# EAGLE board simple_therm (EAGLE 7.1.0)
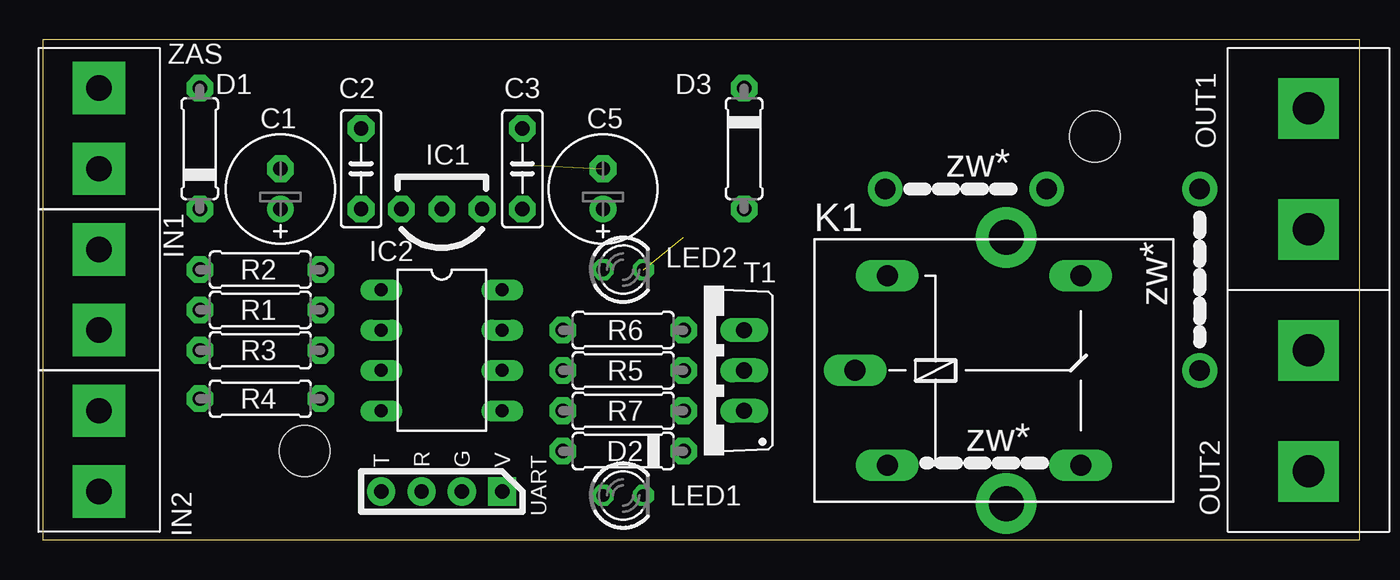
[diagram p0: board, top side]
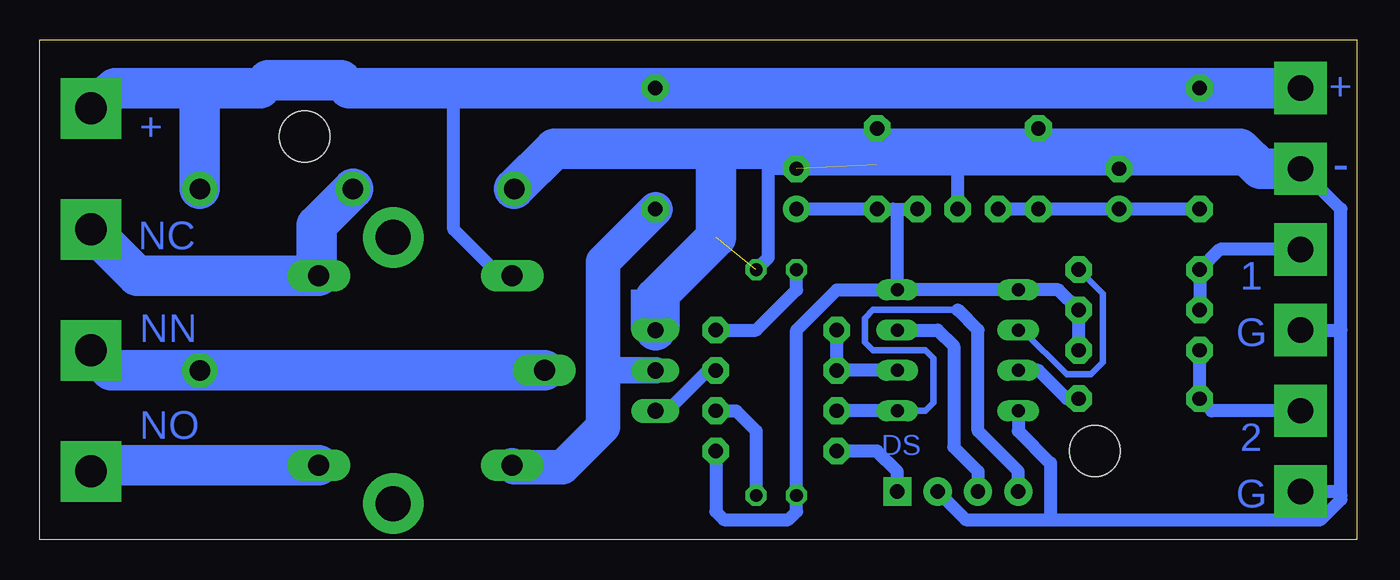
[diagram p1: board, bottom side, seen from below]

Size 82.98 x 31.49 mm. Coordinates in mm from the lower left corner, seen from the top.
Outline: 0,0 82.98,0 82.98,31.49 0,31.49 0,0
Copper layers (1*16): Top 0.035mm / dielectric 1.5mm / Bottom 0.035mm
Design rules "default": minimum track width 10mil, minimum drill 24mil, track to track 8mil, track to pad 8mil, pad to pad 8mil, via to via 8mil, smd to smd 8mil, copper to edge 40mil, drill to drill 8mil, minimum pad ring 10mil, minimum via ring 8mil, stop-mask expansion 4mil, vias tented up to drill 0mil, thermal gap 10mil
Holes 3.2 mm at 16.51,5.59 66.29,25.4

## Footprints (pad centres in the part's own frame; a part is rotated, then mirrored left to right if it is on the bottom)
E2,5-7 = drill 0.9 pad 1.676: + -1.27,0 | drill 0.9 pad 1.676 octagon: - 1.27,0
C050-025X075 = drill 0.9 pad 1.676 octagon: 1 -2.54,0; 2 2.54,0
0207/7 = drill 0.9 pad 1.676 octagon: 1 -3.81,0; 2 3.81,0
DIL08 = drill 0.813 long: 1 -3.81,-3.81; 2 -1.27,-3.81; 3 1.27,-3.81; 4 3.81,-3.81; 5 3.81,3.81; 6 1.27,3.81; 7 -1.27,3.81; 8 -3.81,3.81
ARK2/500 = drill 1.6 pad 3.302 square: 1 -2.54,0; 2 2.54,0
G5LE = drill 1.321 long: 1 -7.493,-5.969; 2 -7.493,5.969; O 4.699,5.969; P -9.525,0; S 4.699,-5.969
LED3MM = drill 0.813 octagon: A -1.27,0; K 1.27,0
ARK2/750 = drill 2 pad 3.81 square: 1 -3.81,0; 2 3.81,0
TO220BV = drill 1.016 long: D 0,-2.54; G -2.54,-2.54; S 2.54,-2.54
MOD09 = drill 0.9 pad 1.778 square: 1 0,-3.81 | drill 0.9 pad 1.778: 2 0,-1.27; 3 0,1.27; 4 0,3.81

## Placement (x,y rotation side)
C1  100uF  [E2,5-7]  14.99,22.1 90 top
C2  100nF  [C050-025X075]  20.07,23.37 90 top
C3  100nF  [C050-025X075]  30.23,23.37 90 top
C5  100uF  [E2,5-7]  35.31,22.1 90 top
D1  1N4007  [0207/7]  9.91,24.64 90 top
D2  1N4007  [0207/7]  36.58,5.59 180 top
D3  1N4007  [0207/7]  44.2,24.64 90 top
IC2  Attiny45  [DIL08]  25.15,11.94 270 top
IN1  ARK2ARK2/500  [ARK2/500]  3.56,15.75 270 top
IN2  ARK2ARK2/500  [ARK2/500]  3.56,5.59 270 top
K1  [G5LE]  60.71,10.67 0 top
LED1  [LED3MM]  36.58,2.79 0 top
LED2  [LED3MM]  36.58,17.02 0 top
OUT1  ARK2  [ARK2/750]  79.76,23.37 90 top
OUT2  ARK2  [ARK2/750]  79.76,8.13 90 top
R1  3k  [0207/7]  13.72,14.48 0 top
R2  3k  [0207/7]  13.72,17.02 0 top
R3  3k  [0207/7]  13.72,11.94 0 top
R4  3k  [0207/7]  13.72,8.89 0 top
R5  3k  [0207/7]  36.58,8.13 0 top
R6  3k  [0207/7]  36.58,13.21 0 top
R7  3k  [0207/7]  36.58,10.67 180 top
T1  N-MOSFET  [TO220BV]  41.66,10.67 90 top
UART  [MOD09]  25.15,3.05 90 top
ZAS  ARK2ARK2/500  [ARK2/500]  3.56,25.91 270 top

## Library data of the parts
C1-C3 C5 D1-D3 R1-R7 = rcl
IC2 = avr-7_2
IN1 IN2 OUT1 OUT2 ZAS = dimmer
K1 = relay; OC_FARNELL: unknown; OC_NEWARK: unknown
LED1 LED2 = led
T1 = transistor-power
UART = dslib_eagle 9_new

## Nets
GND: C1.- C2.2 C3.2 C5.- IC2.4 IN1.2 IN2.2 LED2.K T1.S UART.2 ZAS.2
IN1: IC2.2 R2.2
IN2: IC2.3 R4.2
N$1: K1.O OUT1.1
N$3: D2.2 UART.1
N$4: D3.1 K1.1 T1.D
N$5: IN1.1 R1.1 R2.1
N$6: LED2.A R6.2
N$8: IN2.1 R3.1 R4.1
N$11: LED1.K R5.2
N$14: R7.1 T1.G
N$16: K1.P OUT2.2
N$17: K1.S OUT2.1
OUT: IC2.6 R6.1 R7.2
RST: IC2.1
RX: IC2.7 UART.3
TX: IC2.5 R5.1 UART.4
V+: C1.+ C2.1 D1.1
VCC: D1.2 D3.2 K1.2 OUT1.2 ZAS.1
VDD: C3.1 C5.+ D2.1 IC2.8 LED1.A R1.2 R3.2

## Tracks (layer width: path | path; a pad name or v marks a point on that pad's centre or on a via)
GND  (via drill 1.3 pad 2.18)  (2 unrouted)
  Bottom 0.813: UART.2 24.64,1.27 19.3,1.27 | 19.3,1.27 2.29,1.27 1.02,2.54 1.02,2.79 | 1.02,2.79 1.02,13.21 | 1.02,13.21 1.02,20.83 ZAS.2 C1.- C5.- 37.08,23.37 37.08,17.78 LED2.K | IN1.2 1.02,13.21 | IN2.2 1.27,3.05 1.02,2.79 | IC2.4 21.34,6.86 19.3,4.83 19.3,1.27 | C2.2 20.07,23.37 29.97,23.37 30.23,23.62 C3.2
  Bottom 2.54: ZAS.2 6.1,23.37 7.37,24.64 50.55,24.64 v53.09,22.1 | 40.39,23.37 40.39,19.05 44.2,15.24 T1.S
IN1
  Bottom 0.406: IC2.2 21.08,13.21 18.29,10.41 16.76,10.41 16,11.18 16,15.49 R2.2
IN2
  Bottom 0.813: R4.2 18.29,8.89 20.07,10.67 IC2.3
N$1
  Bottom 2.54: K1.O 76.84,16.64 OUT1.1
N$2  (via drill 2.2 pad 3.81)
  other vias: 60.71,19.05
N$3
  Bottom 0.813: UART.1 28.96,4.32 30.23,5.59 D2.2
N$4
  Bottom 1.676: T1.D 47.5,10.67
  Bottom 2.184: D3.1 47.5,17.53 47.5,10.67 47.5,7.11 50.04,4.57 53.09,4.57 K1.1
N$5
  Bottom 0.813: IN1.1 8.64,18.29 R2.1 R1.1
N$6
  Bottom 0.813: R6.2 37.85,13.21 35.31,15.75 LED2.A
N$7  (via drill 0.9 pad 1.68)
  other vias: 22.61,20.83
N$8
  Bottom 0.813: IN2.1 9.14,8.13 R4.1 R3.1
N$9  (via drill 0.9 pad 1.68)
  other vias: 27.69,20.83
N$10  (via drill 0.9 pad 1.68)
  Bottom 0.813: v25.15,20.83 25.15,23.88
N$11
  Bottom 0.813: R5.2 39.12,8.13 37.85,6.86 LED1.K
N$12
  Bottom 2.54: 65.53,16.76 65.53,19.81 63.25,22.1
N$13  (via drill 1.3 pad 2.18)
  other vias: 63.25,22.1
N$14
  Bottom 0.813: T1.G 43.43,8.13 40.89,10.67 R7.1
N$15  (via drill 2.2 pad 3.81)
  other vias: 60.71,2.29
N$16  (via drill 1.3 pad 2.18)
  Bottom 2.54: K1.P v72.9,10.67 78.49,10.67 OUT2.2
N$17
  Bottom 2.54: K1.S 79.38,4.7 OUT2.1
OUT
  Bottom 0.813: IC2.6 R7.2 R6.1
RX
  Bottom 0.813: IC2.7 26.42,13.21 25.4,12.19 25.4,5.84 23.88,4.32 UART.3
TX
  Bottom 0.406: 25.15,14.48 30.48,14.48 30.99,13.97 30.99,12.45 30.48,11.94 27.18,11.94 26.67,11.43 26.67,8.64 27.18,8.13 IC2.5
  Bottom 0.813: IC2.5 R5.1 | UART.4 21.34,4.32 23.88,6.86 23.88,13.21 25.15,14.48
V+
  Bottom 0.813: D1.1 C1.+ C2.1 22.61,20.83
VCC  (via drill 1.3 pad 2.18)
  Bottom 0.813: K1.2 53.97,16.64 56.9,19.56 56.9,28.45
  Bottom 2.54: 72.9,28.45 69.09,28.45 68.58,28.96 64.01,28.96 63.5,28.45 56.9,28.45 D3.2 42.93,28.45 D1.2 ZAS.1 | 72.9,28.45 78.23,28.45 OUT1.2 | 72.9,28.45 v72.9,22.1
VDD
  Bottom 0.813: IC2.8 32.77,15.75 35.31,13.21 LED1.A 35.31,1.78 35.81,1.27 39.88,1.27 40.39,1.78 D2.1 | R3.2 R1.2 18.8,15.75 IC2.8 | 29.21,20.83 C3.1 C5.+ | 29.21,20.83 27.69,20.83 | IC2.8 28.96,20.57 29.21,20.83
(copper drawn outside any net)
  shapes: Bottom area x1

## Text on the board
Bottom: + | + | - | NC | 1 | NN | G | 2 | NO | DS | G
tPlace: IC1 | zw* | zw* | zw*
